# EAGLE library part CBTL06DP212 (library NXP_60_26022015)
High-performance DisplayPort Gen2 2 : 1 multiplexer AAL Eindhoven MK
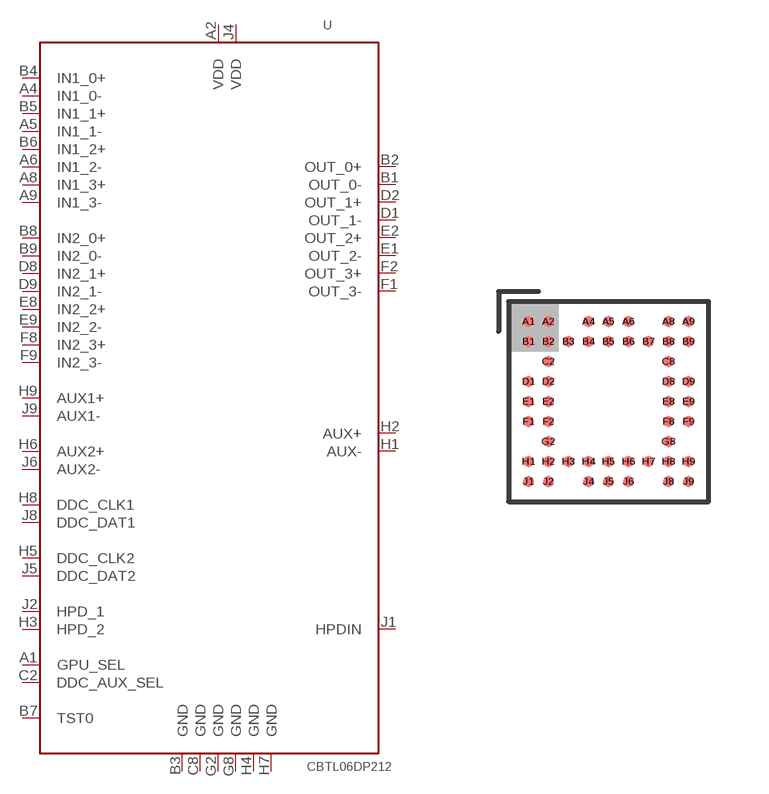
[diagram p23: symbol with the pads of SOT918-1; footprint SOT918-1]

Designator prefix U

## CBTL06DP212  [SOT918-1]
A1  GPU_SEL  in
A2  VDD  pwr
A4  IN1_0-  in
A5  IN1_1-  in
A6  IN1_2-  in
A8  IN1_3+  in
A9  IN1_3-  in
B1  OUT_0-
B2  OUT_0+
B3  GND  pwr
B4  IN1_0+  in
B5  IN1_1+  in
B6  IN1_2+  in
B7  TST0  in
B8  IN2_0+  in
B9  IN2_0-  in
C2  DDC_AUX_SEL  in
C8  GND  pwr
D1  OUT_1-
D2  OUT_1+
D8  IN2_1+  in
D9  IN2_1-  in
E1  OUT_2-
E2  OUT_2+
E8  IN2_2+  in
E9  IN2_2-  in
F1  OUT_3-
F2  OUT_3+
F8  IN2_3+  in
F9  IN2_3-  in
G2  GND  pwr
G8  GND  pwr
H1  AUX-
H2  AUX+
H3  HPD_2  in
H4  GND  pwr
H5  DDC_CLK2  in
H6  AUX2+  in
H7  GND  pwr
H8  DDC_CLK1  in
H9  AUX1+  in
J1  HPDIN  out
J2  HPD_1  in
J4  VDD  pwr
J5  DDC_DAT2  in
J6  AUX2-  in
J8  DDC_DAT1  in
J9  AUX1-  in

## Footprint SOT918-1 (pad centres in mm)
SOT918-1 TFBGA48: plastic thin fine-pitch ball grid array package; 48 balls; body 5 x 5 x 0.8 mm JEDEC: MO-195 IEC: --
smd 0.275 x 0.275: A1 -2,2; A2 -1.5,2; A4 -0.5,2; A5 0,2; A6 0.5,2; A8 1.5,2; A9 2,2; B1 -2,1.5; B2 -1.5,1.5; B3 -1,1.5; B4 -0.5,1.5; B5 0,1.5; B6 0.5,1.5; B7 1,1.5; B8 1.5,1.5; B9 2,1.5; C2 -1.5,1; C8 1.5,1; D1 -2,0.5; D2 -1.5,0.5; D8 1.5,0.5; D9 2,0.5; E1 -2,0; E2 -1.5,0; E8 1.5,0; E9 2,0; F1 -2,-0.5; F2 -1.5,-0.5; F8 1.5,-0.5; F9 2,-0.5; G2 -1.5,-1; G8 1.5,-1; H1 -2,-1.5; H2 -1.5,-1.5; H3 -1,-1.5; H4 -0.5,-1.5; H5 0,-1.5; H6 0.5,-1.5; H7 1,-1.5; H8 1.5,-1.5; H9 2,-1.5; J1 -2,-2; J2 -1.5,-2; J4 -0.5,-2; J5 0,-2; J6 0.5,-2; J8 1.5,-2; J9 2,-2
